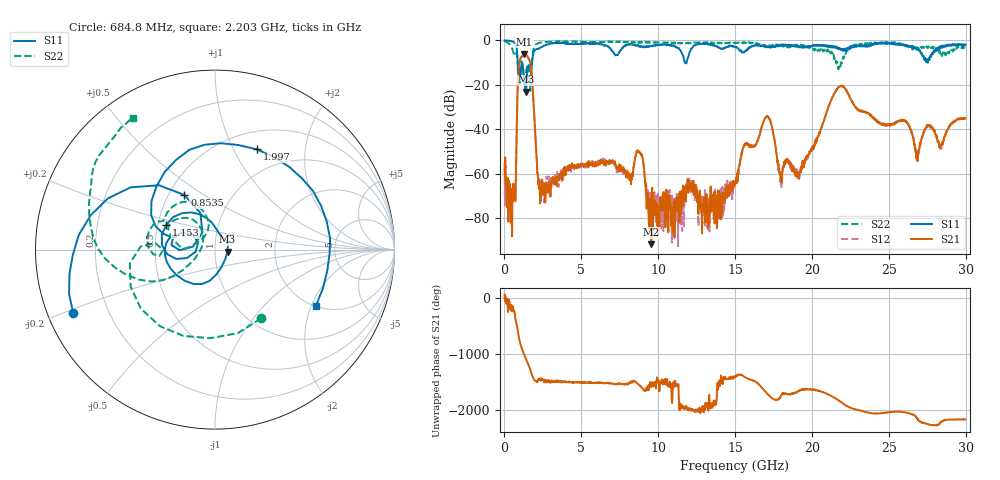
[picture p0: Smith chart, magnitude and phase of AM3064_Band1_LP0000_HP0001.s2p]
# Hz S DB R 50.0
!freq dBS11 angS11 dBS21 angS21 dBS12 angS12 dBS22 angS22
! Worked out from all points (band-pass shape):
!   1600 points, 10 MHz to 29.98 GHz, reference 50 ohm
!   highest |S21| = -6.16 dB at 1.303 GHz (marker M1); lowest = -91.7 dB at 9.551 GHz (marker M2)
!   |S21| within 3 dB of the highest: 999.2 MHz to 1.637 GHz (637.6 MHz wide, 48.4 % of centre)
!   lowest |S11| = -23.0 dB at 1.397 GHz (marker M3), VSWR 1.15, Z = 57.5 - j1.32 ohm
!   |S11| at or under -10 dB: 857.5 MHz to 1.795 GHz (937.6 MHz wide, 70.7 % of centre); 11.74 GHz to 11.85 GHz (104.7 MHz wide, 0.888 % of centre); 27.52466 GHz to 27.53056 GHz (5.892 MHz wide, 0.0214 % of centre)
!   |S22| runs from -22.7 to -0.2 dB; largest |S21 - S12| = 0.0062
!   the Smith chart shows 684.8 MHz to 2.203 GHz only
!   S11 on the Smith chart (normalised r, x): 684.8 MHz: 0.08, -0.21; 853.5 MHz: 0.60, +0.42; 1.153 GHz: 0.55, +0.17; 1.997 GHz: 0.71, +1.24; 2.203 GHz: 2.03, -2.16
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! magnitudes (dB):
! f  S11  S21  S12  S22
! 10 MHz  0.0  -55.7  -57.5  -0.2
! 384.9 MHz  -0.3  -67.1  -66.8  -2.1
! 684.8 MHz  -1.3  -67.3  -71.0  -6.7
! 853.5 MHz  -9.1  -22.8  -22.8  -9.5
! 1.153 GHz  -10.3  -7.1  -7.0  -10.1
! 1.303 GHz  -19.6  -6.2  -6.1  -20.3
! 1.397 GHz  -23.0  -6.4  -6.4  -14.4
! 1.716 GHz  -12.7  -11.5  -11.4  -18.2
! 1.997 GHz  -4.4  -40.9  -40.8  -2.3
! 2.203 GHz  -3.8  -64.7  -64.3  -1.2
! 5.015 GHz  -1.4  -55.8  -56.4  -0.6
! 8.745 GHz  -2.6  -50.4  -49.6  -1.2
! 9.551 GHz  -2.5  -91.7  -70.9  -1.0
! 10 GHz  -2.0  -78.5  -77.1  -0.9
! 15 GHz  -2.9  -65.0  -64.4  -1.2
! 17.05 GHz  -2.8  -34.1  -34.2  -2.7
! 17.97 GHz  -2.4  -63.8  -61.7  -2.1
! 19.99 GHz  -2.8  -48.8  -48.8  -3.4
! 21.85 GHz  -3.6  -20.5  -20.3  -12.2
! 25 GHz  -1.1  -38.0  -38.1  -1.1
! 26.85 GHz  -4.2  -53.8  -51.4  -3.2
! 29.98 GHz  -1.8  -35.1  -34.8  -3.2
